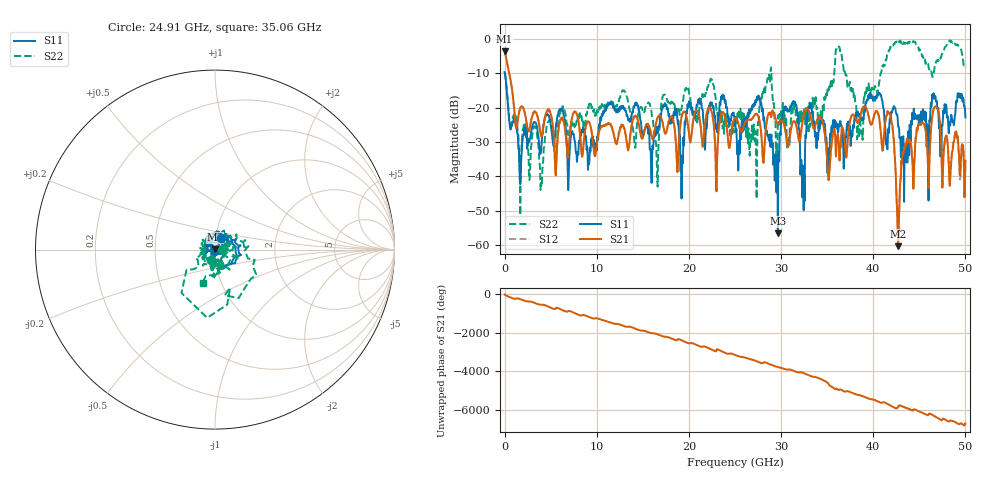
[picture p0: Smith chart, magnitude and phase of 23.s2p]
! 2/2/2024 4:26:46 PM
! D:\_XLC\ZPD9-2M1-50G-2425\23.S2P
! CHANNEL.1
! TR.MEASUREMENT
! CORRECTED.DATA
! RF.CORRECTION: FULL.TWO.PORT.CAL.PORT.1.2
! AVERAGING.OFF
! IF.BANDWIDTH: NO.IFBW
! SWEEPTYPE:  FREQ.SWEEP(Linear)
! Reference Plane Port Info
! PORT:  PORT1  PORT2
! DISTANCE:  0  m  0  m
! TIME:  0  s  0  s
! PHASE.OFFSET:  0 °  0 °
! LOSS:  0  dB  0  dB
! REF.LOSS:  0  dB  0  dB
! REF.FREQ:  0  Hz  0  Hz
! Power Info
! POWER:  0  dBm  0  dBm
! EFF.POWER:  0  dBm  0  dBm
! SOURCE.ATTEN:  0  dB  0  dB
! TEST.ATTEN:  0  dB  0  dB
# GHZ S RI R 50.0
! FREQ.GHZ  S11RE  S11IM  S21RE  S21IM  S12RE  S12IM  S22RE  S22IM
!; PortSelection: Port_12
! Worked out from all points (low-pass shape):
!   1001 points, 10 MHz to 50.01 GHz, reference 50 ohm
!   highest |S21| = -3.64 dB at 10 MHz (marker M1); lowest = -60.4 dB at 42.71 GHz (marker M2)
!   |S21| within 3 dB of the highest: start of sweep to 248.5 MHz
!   lowest |S11| = -56.6 dB at 29.66 GHz (marker M3), VSWR 1.00, Z = 50 + j0.141 ohm
!   |S11| at or under -10 dB: 38.45 MHz to end of sweep
!   |S22| runs from -51.3 to -0.5 dB; largest |S21 - S12| = 0.011
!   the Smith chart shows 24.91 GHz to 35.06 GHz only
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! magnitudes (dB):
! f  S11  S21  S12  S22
! 10 MHz  -9.7  -3.6  -3.6  -9.7
! 1.66 GHz  -41.1  -20.5  -20.5  -38.7
! 3.96 GHz  -32.8  -28.3  -28.3  -41.9
! 8.36 GHz  -26.5  -33.3  -33.3  -22.7
! 12.91 GHz  -20.2  -25.6  -25.4  -15.1
! 16.71 GHz  -25.5  -22.5  -22.5  -31.0
! 17.31 GHz  -19.7  -26.4  -26.5  -16.4
! 22.41 GHz  -19.2  -20.4  -20.7  -11.9
! 25.01 GHz  -22.9  -23.0  -23.1  -23.6
! 27.21 GHz  -18.0  -22.0  -22.1  -26.8
! 28.71 GHz  -29.7  -21.6  -21.6  -10.5
! 29.66 GHz  -56.6  -24.8  -24.8  -23.9
! 31.41 GHz  -18.6  -24.0  -23.8  -20.9
! 32.36 GHz  -36.9  -23.5  -23.7  -21.3
! 33.36 GHz  -21.8  -24.6  -24.6  -20.3
! 36.26 GHz  -24.9  -30.3  -30.6  -2.2
! 38.66 GHz  -23.4  -21.7  -21.8  -26.4
! 41.71 GHz  -27.4  -21.5  -22.2  -3.4
! 42.71 GHz  -25.5  -60.4  -59.1  -1.2
! 43.46 GHz  -35.7  -31.8  -31.9  -1.2
! 46.76 GHz  -16.7  -19.7  -19.9  -7.0
! 50.01 GHz  -22.9  -35.5  -35.2  -8.4
